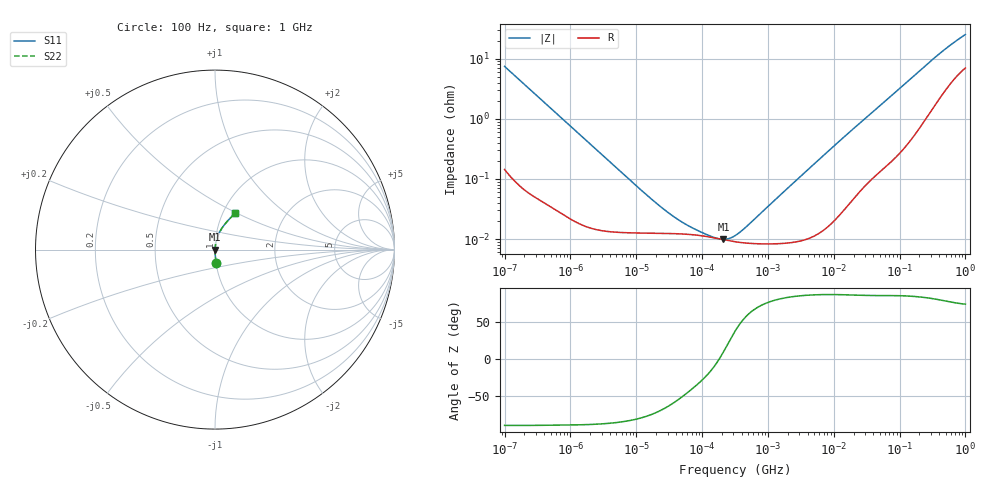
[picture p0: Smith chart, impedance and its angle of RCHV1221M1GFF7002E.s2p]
! RCHV1221M1GFF7002E  S-PARAMETER MODEL  (AEC-Q200 qualified)
! Model Generated by ELNA Corporation (http://www.ty-top.com)
! Version 1.0
! ELNA Control No. 240229
! Copyright (c) 2024 ELNA CO.,LTD. All Rights Reserved.
! Products Name : CONDUCTIVE POLYMER HYBRID ALUMINUM ELECTROLYTIC CAPACITORS
! Characteristics :
!  Capacitance  :  220uF  ,  Rated voltage  :  35V
!  Operating Temp. Range  :  -55 to +105 degC  ,  Endurance  :  10000hr at 105 degC
!  Dimension D  :  10mm  ,  Dimension L  :  8.7mm
! Frequency Range : 100Hz - 1GHz
! External Node Assignments :
!  1  o---| |---o  2
# MHz S RI R 50
!Freq[MHz].  S11 Real  S11 Imag  S21 Real  S21 Imag  S12 Real  S12 Imag  S22 Real  S22 Imag
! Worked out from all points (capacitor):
!   401 points, 100 Hz to 1 GHz, reference 50 ohm
!   read as one part in series: C = 214 uF near 108 Hz
!   lowest |Z| = 9.91 mohm at 211.3 kHz (marker M1)
!   series resonance near 181.6 kHz, so ESL is about 3.6 nH
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0.0001  0.0069 -0.0736  0.9931 0.0736  0.9931 0.0736  0.0069 -0.0736
0.000113  0.00552 -0.0654  0.9945 0.0654  0.9945 0.0654  0.00552 -0.0654
0.000309  0.00106 -0.0241  0.9989 0.0241  0.9989 0.0241  0.00106 -0.0241
0.001488  0.000198 -0.00509  0.9998 0.00509  0.9998 0.00509  0.000198 -0.00509
0.009495  0.000127 -0.0008  0.9999 0.0008  0.9999 0.0008  0.000127 -0.0008
0.022131  0.000125 -0.000342  0.9999 0.000342  0.9999 0.000342  0.000125 -0.000342
0.040504  0.000123 -0.000184  0.9999 0.000184  0.9999 0.000184  0.000123 -0.000184
0.068391  0.000119 -0.000103  0.9999 0.000103  0.9999 0.000103  0.000119 -0.000103
0.141254  0.000107 -2.61e-05  0.9999 2.61e-05  0.9999 2.61e-05  0.000107 -2.61e-05
0.172783  0.000102 -5.34e-06  0.9999 5.34e-06  0.9999 5.34e-06  0.000102 -5.34e-06
0.211349  9.77e-05 1.7e-05  0.9999 -1.7e-05  0.9999 -1.7e-05  9.77e-05 1.7e-05
0.258523  9.37e-05 4.16e-05  0.9999 -4.16e-05  0.9999 -4.16e-05  9.37e-05 4.16e-05
0.316228  9.04e-05 6.93e-05  0.9999 -6.93e-05  0.9999 -6.93e-05  9.04e-05 6.93e-05
0.371535  8.82e-05 9.41e-05  0.9999 -9.41e-05  0.9999 -9.41e-05  8.82e-05 9.41e-05
0.473151  8.59e-05 0.000137  0.9999 -0.000137  0.9999 -0.000137  8.59e-05 0.000137
4.704354  0.000111 0.00165  0.9999 -0.00165  0.9999 -0.00165  0.000111 0.00165
16.4059  0.000394 0.00567  0.9996 -0.00567  0.9996 -0.00567  0.000394 0.00567
69.9842  0.00231 0.0224  0.9977 -0.0224  0.9977 -0.0224  0.00231 0.0224
169.8244  0.00814 0.0524  0.9919 -0.0524  0.9919 -0.0524  0.00814 0.0524
380.1894  0.0311 0.1071  0.9689 -0.1071  0.9689 -0.1071  0.0311 0.1071
641.9482  0.067 0.1561  0.933 -0.1561  0.933 -0.1561  0.067 0.1561
1000  0.1109 0.2013  0.8891 -0.2013  0.8891 -0.2013  0.1109 0.2013
